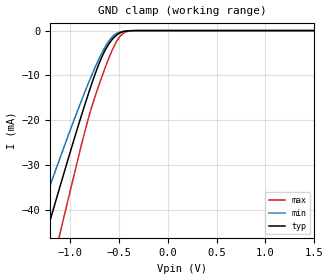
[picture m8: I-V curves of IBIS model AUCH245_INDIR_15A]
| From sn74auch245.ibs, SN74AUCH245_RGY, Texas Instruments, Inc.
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[Model]   AUCH245_INDIR_15A
Model_type  Input
Vinl=0.49
Vinh=1.04
| variable   typ   min   max
C_comp   2.57pF   2.10pF   3.01pF
[Temperature Range]   40   100   -40
| Ambient temperature   25   85   -40
[Voltage range]   1.5   1.4   1.6
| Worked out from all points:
|   GND clamp passes 1 mA (typ) near -0.52 V on its own axis
[GND Clamp]
| AUCH245_INDIR_15A
|   Voltage   I(typ)   I(min)   I(max)
-3.6V     -229.3mA   -192.6mA   -273mA
-1.365V   -54.68mA   -44.68mA   -69.45mA
-1.23V    -44.43mA   -36.28mA   -57.06mA
-1.11V    -35.45mA   -28.97mA   -46.07mA
-1.065V   -32.12mA   -26.27mA   -41.97mA
-815mV    -14.38mA   -11.99mA   -19.92mA
-700mV    -7.296mA   -6.219mA   -11.99mA
-585mV    -2.484mA   -1.884mA   -5.281mA
-515mV    -880.3uA   -569.4uA   -2.161mA
-460mV    -279.4uA   -178.2uA   -714.3uA
-315mV    -4.754uA   -4.767uA   -5.622uA
1.5V      253.5pA    827.7pA    37.14pA
